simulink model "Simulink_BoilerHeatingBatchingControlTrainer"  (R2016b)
settings: Solver=VariableStepAuto  StartTime=0.0  StopTime=10000  RelTol=1e-3
libraries: simulink x28, sldrtlib x1
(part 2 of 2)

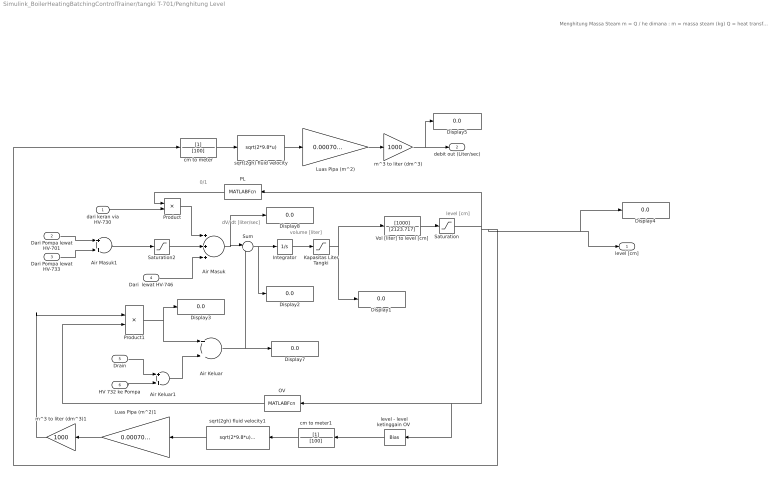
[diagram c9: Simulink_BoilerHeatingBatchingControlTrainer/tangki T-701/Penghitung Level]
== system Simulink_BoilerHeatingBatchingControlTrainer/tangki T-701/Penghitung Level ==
  note: 0/1
  note: dV/ dt [liter/sec]
  note: level [cm]
  note: volume [liter]
  note: Menghitung Massa Steam m = Q / he dimana : m = massa steam (kg) Q = heat transfer (J) he = Spesific laten heat evaporation (J/kg)
  dari keran via HV-730 : Inport  RequirementInfo={} %GIDa_58f6ba86_5855_4df4_bf99_0f9320cae496
  Dari Pompa lewat HV-701 : Inport  RequirementInfo={} %GIDa_c6417745_8917_411c_9690_2e3c100096b9  Port=2
  Dari Pompa lewat HV-733 : Inport  RequirementInfo={} %GIDa_3f0d2854_948f_4fdc_a9be_e73e1e9b4dcf  Port=3
  Dari  lewat HV-746 : Inport  RequirementInfo={} %GIDa_242d4b19_598a_44bb_8fe6_af30078015c8  Port=4
  Drain : Inport  RequirementInfo={} %GIDa_0358b676_d126_4230_8c20_fc59f125fd8d  Port=5
  HV 732 ke Pompa : Inport  RequirementInfo={} %GIDa_a100b2f0_83be_4d5a_9135_17066da4f5b6  Port=6
  Air Keluar : Sum  RequirementInfo={} %GIDa_9c07271b_d687_4b7f_8e01_1b69ebb3a752
  Air Keluar1 : Sum  RequirementInfo={} %GIDa_566d9eeb_9954_4dc7_9436_c118a183d389
  Air Masuk : Sum  RequirementInfo={} %GIDa_d7462d81_6a29_466a_b502_53ee4915dc24  Inputs=+++
  Air Masuk1 : Sum  RequirementInfo={} %GIDa_beb8bcd2_7b4c_4095_97f8_cfb909a72fa8
  Display{1..5,7..8} (7 alike) : Display
  Integrator : Integrator  RequirementInfo={} %GIDa_f30a5aec_56d5_4116_8f53_9258476a2796
  Kapasitas Liter Tangki : Saturate  RequirementInfo={} %GIDa_85cbc076_33d9_4412_a394_8cf7bc203153  UpperLimit=120  LowerLimit=-99999999999999999999999999999999999999999999999999999999
  Luas Pipa (m^2) : Gain  RequirementInfo={} %GIDa_0e09d8b1_07b8_4f90_9b19_64c10180463a  Gain=0.000706858347
  Luas Pipa (m^2)1 : Gain  RequirementInfo={} %GIDa_0864a421_17e2_476e_951e_723b80871d8e  Gain=0.000706858347
  OV : MATLABFcn  RequirementInfo={} %GIDa_385466d3_94cd_41f9_baf1_63d7178c01c5  MATLABFcn=OV
  PL : MATLABFcn  RequirementInfo={} %GIDa_824498d7_3bc8_4ec7_8282_8c412cc74980  MATLABFcn=PL
  Product : Product  RequirementInfo={} %GIDa_384d461e_f373_44c8_be57_dd7a2638b7c3
  Product1 : Product  RequirementInfo={} %GIDa_5f7b7aa2_d3e6_4aba_9f15_33d105d3af69
  Saturation : Saturate  RequirementInfo={} %GIDa_081c38eb_98f7_4fd3_a150_48f9722132cc  UpperLimit=65.5  LowerLimit=0
  Saturation2 : Saturate  RequirementInfo={} %GIDa_d66e23e9_fa49_498b_a495_352d197f1182  UpperLimit=1  LowerLimit=-999999999999999999999999999999999999999999999999999999
  Sum : Sum  RequirementInfo={} %GIDa_032508b3_ec76_4eb1_81af_7ae6fc921670  Inputs=|+-
  Vol [liter] to level [cm] : TransferFcn  RequirementInfo={} %GIDa_b64f84bb_97c5_4b40_8195_27d14b33ccde  Numerator=[1000]  Denominator=[2123.717]
  cm to meter : TransferFcn  RequirementInfo={} %GIDa_f2625284_93f4_463e_8081_ad992fa8cafd  Denominator=[100]
  cm to meter1 : TransferFcn  RequirementInfo={} %GIDa_fc5c7aab_fe04_4522_91b1_85e6ba885d2c  Denominator=[100]
  "level - level ketinggain OV " : Bias  RequirementInfo={} %GIDa_b853cae0_bff0_4c1a_bb6d_d914c2536c45  Bias=-60
  m^3 to liter (dm^3) : Gain  RequirementInfo={} %GIDa_d72bbef3_c132_4bb2_9fd7_70e611914f57  Gain=1000
  m^3 to liter (dm^3)1 : Gain  RequirementInfo={} %GIDa_00183f06_5c63_4ed9_8a4f_bdef8bc6cd9f  Gain=1000
  sqrt(2gh) fluid velocity : Fcn  RequirementInfo={} %GIDa_83a942a7_e023_4c66_b2bd_d0ee91fdf5a6  Expr=sqrt(2*9.8*u)
  sqrt(2gh) fluid velocity1 : Fcn  RequirementInfo={} %GIDa_31d0e8d2_89a4_40f0_a049_be62e84a6d20  Expr=sqrt(2*9.8*u)+0.00001
  level [cm] : Outport  RequirementInfo={} %GIDa_13b721a9_06b3_45e9_b636_0e20b7beb282
  debit out (Liter/sec) : Outport  RequirementInfo={} %GIDa_cb85f3f9_8c7a_49f2_88ac_d52dfae9f33b  Port=2
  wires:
  Vol [liter] to level [cm]/1 -> Saturation/1
  Integrator/1 -> Kapasitas Liter Tangki/1
  Sum/1 -> Integrator/1, Display2/1
  Air Masuk/1 -> Display8/1, Sum/1
  Dari  lewat HV-746/1 -> Air Masuk/3
  Product/1 -> Air Masuk/1
  dari keran via HV-730/1 -> Product/2
  PL/1 -> Product/1
  m^3 to liter (dm^3)1/1 -> Product1/1
  OV/1 -> Product1/2
  Product1/1 -> Display3/1, Air Keluar/1
  Drain/1 -> Air Keluar1/1
  HV 732 ke Pompa/1 -> Air Keluar1/2
  Air Keluar1/1 -> Air Keluar/2
  Air Keluar/1 -> Display7/1, Sum/2
  m^3 to liter (dm^3)/1 -> Display5/1, debit out (Liter/sec)/1
  sqrt(2gh) fluid velocity/1 -> Luas Pipa (m^2)/1
  Luas Pipa (m^2)/1 -> m^3 to liter (dm^3)/1
  cm to meter/1 -> sqrt(2gh) fluid velocity/1
  cm to meter1/1 -> sqrt(2gh) fluid velocity1/1
  sqrt(2gh) fluid velocity1/1 -> Luas Pipa (m^2)1/1
  Luas Pipa (m^2)1/1 -> m^3 to liter (dm^3)1/1
  "level - level ketinggain OV "/1 -> cm to meter1/1
  Dari Pompa lewat HV-733/1 -> Air Masuk1/2
  Dari Pompa lewat HV-701/1 -> Air Masuk1/1
  Air Masuk1/1 -> Saturation2/1
  Saturation2/1 -> Air Masuk/2
  Kapasitas Liter Tangki/1 -> Vol [liter] to level [cm]/1, Display1/1
  Saturation/1 -> "level - level ketinggain OV "/1, OV/1, Display4/1, level [cm]/1, cm to meter/1, PL/1

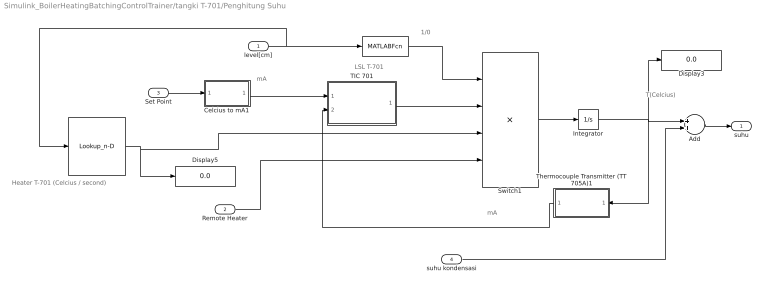
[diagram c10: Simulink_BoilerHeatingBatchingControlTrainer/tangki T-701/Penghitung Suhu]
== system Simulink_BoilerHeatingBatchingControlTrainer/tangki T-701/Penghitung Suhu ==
  note: Heater T-701 (Celcius / second)
  note: mA
  note: mA
  note: T(Celcius)
  note: LSL T-701
  note: 1/0
  level[cm] : Inport  RequirementInfo={} %GIDa_74153236_82a8_472e_9c9d_380c36cfb480
  Remote Heater : Inport  RequirementInfo={} %GIDa_b2b2d110_ce6c_409a_9ef6_42c663c2fb04  Port=2
  Set Point : Inport  RequirementInfo={} %GIDa_f696b8ac_9f02_42ae_b9a3_3966d99664bf  Port=3
  suhu kondensasi : Inport  Port=4
  " " : MATLABFcn  RequirementInfo="{'linktype_rmi_simulink' 'D' ':376' 'true' 'D/Lamp  (SubSystem)' '' } %GIDa_e0a9c92d_26e6_4234_83b3_6e0a329ee748"  MATLABFcn=LSL
  . : Lookup_n-D  NumberOfTableDimensions=1  BreakpointsForDimension1=[30,40,50]  Table=[0.068311,0.054088,0.042156]  InternalRulePriority=Speed  RndMeth=Simplest
  Add : Sum
  Celcius to mA1 : Subsystem  RequirementInfo={} %GIDa_6a115737_0a2d_4fda_9a87_fd6056a1518c
  Display3 : Display
  Display5 : Display
  Integrator : Integrator  RequirementInfo={} %GIDa_5c588f51_8996_453d_959e_029885d3b8ff  InitialCondition=28
  Switch1 : Product  RequirementInfo={} %GIDa_2e270a18_bb40_45e2_97f3_c320fc786cf5  Inputs=4
  TIC 701 : Subsystem  RequirementInfo={} %GIDa_c5d0fefa_df96_4352_b57b_67aebaee03b4
  Thermocouple Transmitter (TT 705A)1 : Subsystem  RequirementInfo={} %GIDa_c60487de_82c8_4118_9995_76d8cfc7fd22
  suhu : Outport  RequirementInfo={} %GIDa_96094640_6a13_425c_b28c_b8cb469993f4
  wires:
  Switch1/1 -> Integrator/1
  Remote Heater/1 -> Switch1/4
  TIC 701/1(Out1) -> Switch1/2
  " "/1 -> Switch1/1
  ./1 -> Display5/1, Switch1/3
  Thermocouple Transmitter (TT 705A)1/1(Out1) -> TIC 701/2(In2)
  Set Point/1 -> Celcius to mA1/1(In1)
  Celcius to mA1/1(Out1) -> TIC 701/1(In1)
  level[cm]/1 -> ./1, " "/1
  Integrator/1 -> Display3/1, Add/1, Thermocouple Transmitter (TT 705A)1/1(In1)
  Add/1 -> suhu/1
  suhu kondensasi/1 -> Add/2

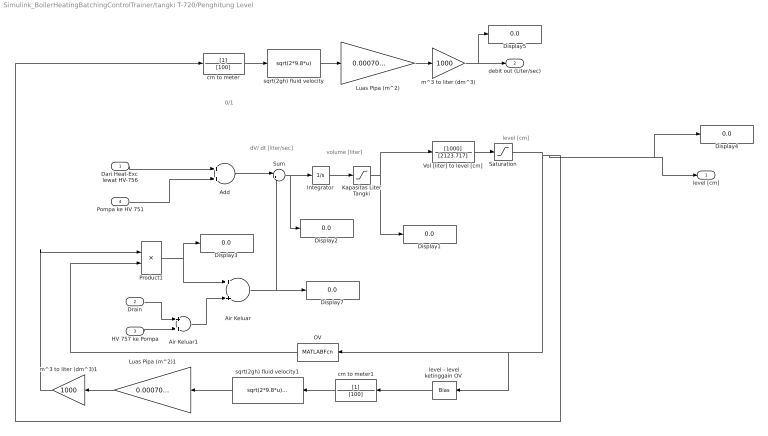
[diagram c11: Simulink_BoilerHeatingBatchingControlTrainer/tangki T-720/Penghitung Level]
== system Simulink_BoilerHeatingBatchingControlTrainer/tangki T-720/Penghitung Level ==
  note: 0/1
  note: dV/ dt [liter/sec]
  note: level [cm]
  note: volume [liter]
  Dari Heat-Exc  lewat HV-756 : Inport  RequirementInfo={} %GIDa_d3d3b0b4_2308_4a5d_82be_64a74fd6ef76
  Drain : Inport  RequirementInfo={} %GIDa_515198cb_bfdb_452a_a343_0988bce7e1a0  Port=2
  HV 757 ke Pompa : Inport  RequirementInfo={} %GIDa_260e0a9f_6abd_4ce6_8705_d7fa409196de  Port=3
  Pompa ke HV 751 : Inport  Port=4
  Add : Sum
  Air Keluar : Sum  RequirementInfo={} %GIDa_ccb87506_c0f2_4266_a756_a567cd7d351e
  Air Keluar1 : Sum  RequirementInfo={} %GIDa_f4027b3e_f995_449c_a825_befb440109df
  Display{1..5,7} (6 alike) : Display
  Integrator : Integrator  RequirementInfo={} %GIDa_6c5e47a1_d0dc_4a4f_b1dd_055b58f653ab
  Kapasitas Liter Tangki : Saturate  RequirementInfo={} %GIDa_300dc90a_a9a3_47d6_b543_fb1ce070a064  UpperLimit=120  LowerLimit=-99999999999999999999999999999999999999999999999999999999
  Luas Pipa (m^2) : Gain  RequirementInfo={} %GIDa_ae18ecb4_e0be_4057_a4eb_a81a59969279  Gain=0.000706858347
  Luas Pipa (m^2)1 : Gain  RequirementInfo={} %GIDa_35ee685d_3e65_4acc_baa9_73c31ce69db5  Gain=0.000706858347
  OV : MATLABFcn  RequirementInfo={} %GIDa_da9b56a3_9a2a_48a7_bd6e_e98e2c1bd977  MATLABFcn=OV
  Product1 : Product  RequirementInfo={} %GIDa_1db03212_3d1f_4403_8ff2_ed9c09fab536
  Saturation : Saturate  RequirementInfo={} %GIDa_1fe0e208_867a_411d_8d03_838fcee455d3  UpperLimit=65.5  LowerLimit=0
  Sum : Sum  RequirementInfo={} %GIDa_622e7568_199f_4634_afc9_9aee7e775c0e  Inputs=|+-
  Vol [liter] to level [cm] : TransferFcn  RequirementInfo={} %GIDa_a9d36b6f_9409_4063_8d68_c397d8246b93  Numerator=[1000]  Denominator=[2123.717]
  cm to meter : TransferFcn  RequirementInfo={} %GIDa_3244f903_3cff_4b71_aaf7_50065633a20c  Denominator=[100]
  cm to meter1 : TransferFcn  RequirementInfo={} %GIDa_b87a6205_7dab_4e75_ad47_a1469aa1ef70  Denominator=[100]
  "level - level ketinggain OV " : Bias  RequirementInfo={} %GIDa_15339c0c_07f6_4326_871f_8e65ec7097ae  Bias=-60
  m^3 to liter (dm^3) : Gain  RequirementInfo={} %GIDa_314b4331_ce17_412c_a601_a1e71d76640b  Gain=1000
  m^3 to liter (dm^3)1 : Gain  RequirementInfo={} %GIDa_b7e6f3d1_ec03_4ca7_8dec_eb2635602ecf  Gain=1000
  sqrt(2gh) fluid velocity : Fcn  RequirementInfo={} %GIDa_747c740a_4c6a_4746_99de_7907750b8506  Expr=sqrt(2*9.8*u)
  sqrt(2gh) fluid velocity1 : Fcn  RequirementInfo={} %GIDa_e5d7118a_598c_4d7c_a12b_21bc606aebae  Expr=sqrt(2*9.8*u)+0.00001
  level [cm] : Outport  RequirementInfo={} %GIDa_94f8bd1e_c9ea_481c_b1c1_fec5a7885fc4
  debit out (Liter/sec) : Outport  RequirementInfo={} %GIDa_d107e7f3_5d61_4fed_a2e6_371d9983ce2e  Port=2
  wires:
  Vol [liter] to level [cm]/1 -> Saturation/1
  Integrator/1 -> Kapasitas Liter Tangki/1
  Sum/1 -> Integrator/1, Display2/1
  m^3 to liter (dm^3)1/1 -> Product1/1
  OV/1 -> Product1/2
  Product1/1 -> Display3/1, Air Keluar/1
  Drain/1 -> Air Keluar1/1
  HV 757 ke Pompa/1 -> Air Keluar1/2
  Air Keluar1/1 -> Air Keluar/2
  Air Keluar/1 -> Display7/1, Sum/2
  m^3 to liter (dm^3)/1 -> Display5/1, debit out (Liter/sec)/1
  sqrt(2gh) fluid velocity/1 -> Luas Pipa (m^2)/1
  Luas Pipa (m^2)/1 -> m^3 to liter (dm^3)/1
  cm to meter/1 -> sqrt(2gh) fluid velocity/1
  cm to meter1/1 -> sqrt(2gh) fluid velocity1/1
  sqrt(2gh) fluid velocity1/1 -> Luas Pipa (m^2)1/1
  Luas Pipa (m^2)1/1 -> m^3 to liter (dm^3)1/1
  "level - level ketinggain OV "/1 -> cm to meter1/1
  Kapasitas Liter Tangki/1 -> Vol [liter] to level [cm]/1, Display1/1
  Saturation/1 -> "level - level ketinggain OV "/1, OV/1, Display4/1, level [cm]/1, cm to meter/1
  Dari Heat-Exc  lewat HV-756/1 -> Add/1
  Add/1 -> Sum/1
  Pompa ke HV 751/1 -> Add/2

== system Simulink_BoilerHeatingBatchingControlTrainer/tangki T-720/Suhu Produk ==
  Suhu T-720 : Inport
  Suhu. T-720 : Outport
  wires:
  Suhu T-720/1 -> Suhu. T-720/1

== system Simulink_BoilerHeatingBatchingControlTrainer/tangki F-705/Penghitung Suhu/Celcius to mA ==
  In1 : Inport  RequirementInfo={} %GIDa_db6e118d_8833_4c3b_a629_8f4447b1ac0e
  Add : Sum  RequirementInfo={} %GIDa_ca6bff12_9a5b_418d_a13f_80a78a609940
  initial condition (mA) : Constant  RequirementInfo={} %GIDa_6b554928_76ac_41d6_8045_5c3d6b5566e9  Value=4
  to mA : Gain  RequirementInfo={} %GIDa_43c00303_9561_4c4b_b603_69e823da6160  Gain=0.16
  Out1 : Outport  RequirementInfo={} %GIDa_c1574f33_1683_4536_85c2_e2757caa2a23
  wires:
  In1/1 -> to mA/1
  to mA/1 -> Add/1
  Add/1 -> Out1/1
  initial condition (mA)/1 -> Add/2

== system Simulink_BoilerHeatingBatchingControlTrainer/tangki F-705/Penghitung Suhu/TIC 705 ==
  note: 1/0
  In2 : Inport  RequirementInfo={} %GIDa_49572ced_ac8b_49bf_a994_df4b37b59533
  In3 : Inport  RequirementInfo={} %GIDa_c5b0a742_d5c2_42fc_b86d_83ee653e6c2c  Port=2
  ON/OFF Controller : MATLABFcn  RequirementInfo={} %GIDa_269f0e47_ca39_4ada_81cf_e5c24e422869  MATLABFcn=TM
  Sum1 : Sum  RequirementInfo={} %GIDa_ab33311e_a034_4b7f_a945_4cb6bf470606  Inputs=|+-
  Out1 : Outport  RequirementInfo={} %GIDa_c1226823_362c_4f77_8981_81c090200e2a
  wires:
  In3/1 -> Sum1/2
  Sum1/1 -> ON/OFF Controller/1
  In2/1 -> Sum1/1
  ON/OFF Controller/1 -> Out1/1

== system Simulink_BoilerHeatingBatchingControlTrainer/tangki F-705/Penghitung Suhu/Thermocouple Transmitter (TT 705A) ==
  In2 : Inport  RequirementInfo={} %GIDa_e9f345ea_79b5_4ca1_bf58_ffeb9b043c64
  Bias : Bias  RequirementInfo={} %GIDa_724471aa_ff49_453a_b9d5_f91526014c9d  Bias=4
  Thermocouple Sensor : TransferFcn  RequirementInfo={} %GIDa_c8360ada_dd26_4d96_84e0_4c60127da8da  Numerator=[0.16]  Denominator=[1 1]
  Out2 : Outport  RequirementInfo={} %GIDa_ccba9003_0a2e_44c0_b134_95bd3ff4a8f2
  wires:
  Bias/1 -> Out2/1
  In2/1 -> Thermocouple Sensor/1
  Thermocouple Sensor/1 -> Bias/1

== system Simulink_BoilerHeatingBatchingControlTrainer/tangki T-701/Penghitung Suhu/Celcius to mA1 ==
  In1 : Inport  RequirementInfo={} %GIDa_a96f1743_a6ee_43a4_9bed_ff6a31d266f1
  Add : Sum  RequirementInfo={} %GIDa_08fcc59a_3a93_4592_9186_ecbc0d32d834
  initial condition (mA) : Constant  RequirementInfo={} %GIDa_e6ea8f86_9047_4fc5_8482_b50284623dbd  Value=4
  to mA : Gain  RequirementInfo={} %GIDa_279cff82_4cb1_4897_a866_b5c7f42ff3dd  Gain=0.16
  Out1 : Outport  RequirementInfo={} %GIDa_2e62fa72_dead_4d43_91eb_67dba7358719
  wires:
  In1/1 -> to mA/1
  to mA/1 -> Add/1
  Add/1 -> Out1/1
  initial condition (mA)/1 -> Add/2

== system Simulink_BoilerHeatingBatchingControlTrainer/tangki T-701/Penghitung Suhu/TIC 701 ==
  note: 1/0
  In1 : Inport  RequirementInfo={} %GIDa_db5afd6a_500e_480c_a557_458815a32f3e
  In2 : Inport  RequirementInfo={} %GIDa_babf0f97_1346_47ef_986d_2d22512604de  Port=2
  ON/OFF Controller : MATLABFcn  RequirementInfo={} %GIDa_820f602d_765b_47b9_8aa0_9370bad726e3  MATLABFcn=TM
  Sum1 : Sum  RequirementInfo={} %GIDa_d8eff442_cdff_448c_9cd4_0d7eedff05ed  Inputs=|+-
  Out1 : Outport  RequirementInfo={} %GIDa_786692c9_9dd9_4892_9e15_c338071608c8
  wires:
  In2/1 -> Sum1/2
  Sum1/1 -> ON/OFF Controller/1
  In1/1 -> Sum1/1
  ON/OFF Controller/1 -> Out1/1

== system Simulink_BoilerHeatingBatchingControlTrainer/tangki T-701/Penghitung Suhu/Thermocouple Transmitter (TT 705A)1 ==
  note: mA
  In1 : Inport  RequirementInfo={} %GIDa_b81dbb7f_3012_42d0_9512_fe1d7243d064
  Bias : Bias  RequirementInfo={} %GIDa_69a1cbd1_aa26_4599_9ed9_57e2cab19984  Bias=4
  Thermocouple Transmitter Transfer Function : TransferFcn  RequirementInfo={} %GIDa_36be528f_58ef_46e1_b4a1_5ee68935b1f3  Numerator=[0.16]  Denominator=[2 1]
  Out1 : Outport  RequirementInfo={} %GIDa_f1f2c72f_cf8e_42bd_80f9_ae9c594188c4
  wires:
  Bias/1 -> Out1/1
  In1/1 -> Thermocouple Transmitter Transfer Function/1
  Thermocouple Transmitter Transfer Function/1 -> Bias/1
